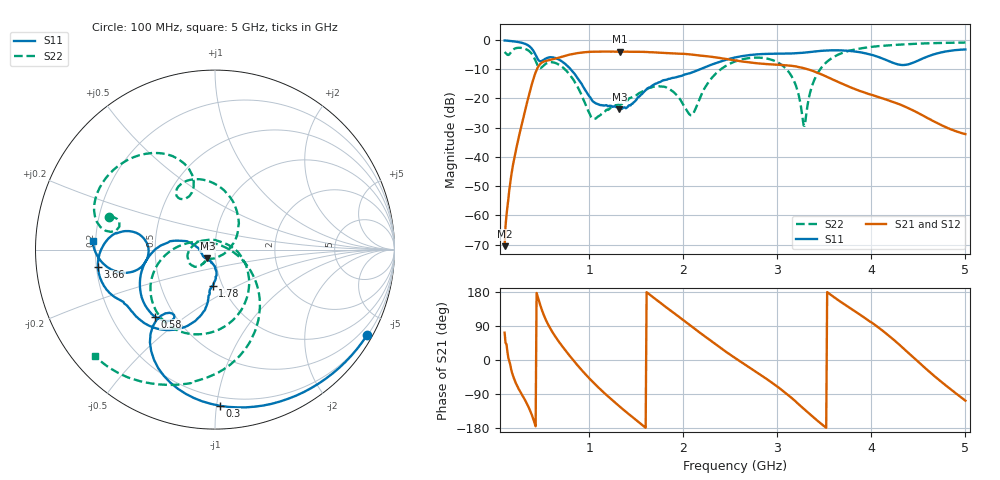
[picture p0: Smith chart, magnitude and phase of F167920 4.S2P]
!  2-Port S-parameters saved by WinCal
! VAR MeasName=S-Parameters (CALIBRATED_DATA) read from VNA (N5242A)
! VAR MeasDate=2016-11-22 9:53:35
! VAR NAME=F167920 4
! VAR FILENAME=F167920 4.S2P
! VAR DATE=2016-11-22 9:53:35
! VAR PHYS_PORTS=1,2
# Hz S DB R 50
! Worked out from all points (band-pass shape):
!   491 points, 100 MHz to 5 GHz, reference 50 ohm
!   highest |S21| = -4.02 dB at 1.33 GHz (marker M1); lowest = -70.5 dB at 100 MHz (marker M2)
!   |S21| within 3 dB of the highest: 566.4 MHz to 2.539 GHz (1.973 GHz wide, 127 % of centre)
!   lowest |S11| = -23.8 dB at 1.32 GHz (marker M3), VSWR 1.14, Z = 45.7 - j4.48 ohm
!   |S11| at or under -10 dB: 800.6 MHz to 2.185 GHz (1.385 GHz wide, 92.8 % of centre)
!   |S22| runs from -29.4 to -1.0 dB; largest |S21 - S12| = 0.0016
!   S11 on the Smith chart (normalised r, x): 100 MHz: 0.22, -3.82; 300 MHz: 0.14, -1.02; 580 MHz: 0.39, -0.39; 1.78 GHz: 0.90, -0.38; 3.66 GHz: 0.21, -0.07; 5 GHz: 0.19, +0.03
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1e8  -0.25 -29.3  -70.47 72.2  -69.12 44.7  -4.19 162.7
1.8e8  -0.50 -52.2  -44.47 -34.4  -44.48 -34.8  -3.74 168.9
3e8  -1.20 -88.2  -26.50 -98.2  -26.50 -98.2  -2.93 139.3
4.6e8  -6.94 -127.9  -9.06 160.3  -9.05 160.4  -9.26 111.8
5.8e8  -5.98 -132.1  -6.90 85.6  -6.89 85.6  -7.68 116.4
7.7e8  -9.00 -176.6  -5.27 18.0  -5.26 17.9  -11.05 68.1
9.2e8  -15.09 164.2  -4.34 -26.5  -4.34 -26.5  -19.11 19.6
1.05e9  -21.30 -178.5  -4.10 -61.1  -4.10 -61.1  -27.04 -62.7
1.32e9  -23.77 -131.1  -4.02 -121.8  -4.02 -121.8  -22.16 -134.4
1.33e9  -23.72 -126.8  -4.02 -124.1  -4.02 -124.1  -22.21 -132.4
1.74e9  -14.53 -92.1  -4.42 154.0  -4.41 154.0  -15.86 -156.8
1.78e9  -13.94 -93.4  -4.46 146.3  -4.45 146.4  -16.00 -163.1
2.09e9  -11.19 -97.7  -5.06 88.0  -5.05 88.0  -25.78 66.0
2.3e9  -8.51 -102.2  -5.81 49.3  -5.81 49.3  -13.16 -33.7
2.55e9  -6.06 -116.4  -7.07 5.4  -7.06 5.4  -7.44 -81.0
3.07e9  -4.74 -145.6  -8.67 -83.4  -8.65 -83.5  -9.21 -162.8
3.19e9  -4.62 -149.2  -9.06 -108.2  -9.04 -108.3  -15.01 170.5
3.28e9  -4.43 -152.1  -9.70 -128.4  -9.67 -128.6  -29.25 92.0
3.37e9  -4.11 -155.5  -10.57 -148.1  -10.54 -148.3  -15.68 -20.9
3.66e9  -3.62 -171.4  -14.63 155.8  -14.62 155.6  -4.91 -71.7
4.19e9  -7.37 168.8  -20.78 63.2  -20.81 63.2  -1.89 -110.4
5e9  -3.31 176.2  -32.23 -107.3  -32.26 -107.6  -0.97 -138.4
